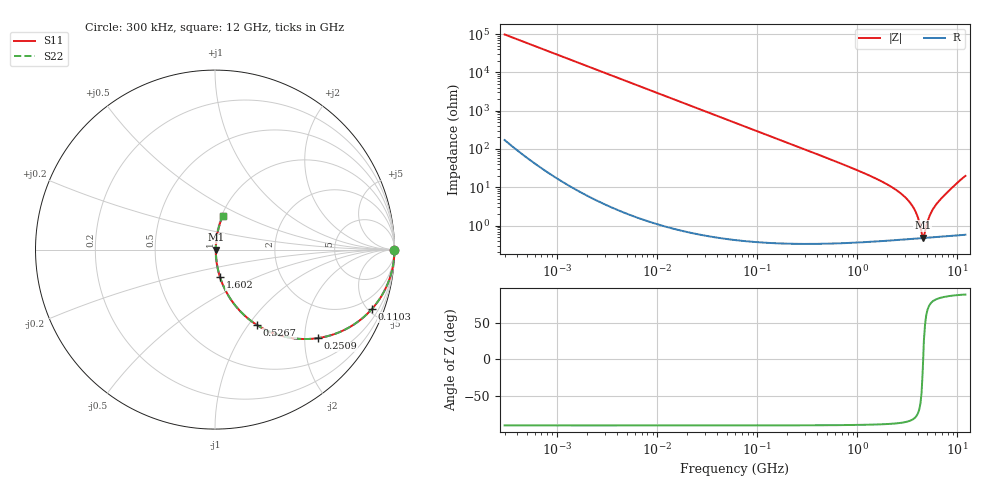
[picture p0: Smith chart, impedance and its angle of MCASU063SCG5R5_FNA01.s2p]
! MCASU063SCG5R5_FNA01  S-PARAMETER MODEL  ( General Type )
! Model Generated by TAIYO YUDEN Corporation (http://www.ty-top.com)
! Version 1.0
! TAIYO YUDEN Control No. 130801
! Copyright(c) 2013 TAIYO YUDEN CO.,LTD. All Rights Reserved.
! Product Description (link to TY-COMPAS)
! https://ds.yuden.co.jp/TYCOMPAS/or/detail?pn=MCASU063SCG5R5DFNA01&u=M
! Products Name : Multilayer Ceramic Capacitors
! Characteristics :
!  Capacitance : 5.5 pF , Rated Voltage : 50V , TCC : CG / C0G
!  Case Size : 0.6 x 0.3 / 0.024 x 0.012 [mm/inch] , Thickness : 0.3 / 0.012 [mm/inch]
!  (Conditions: Temperature = 25 degC , DC Bias Current/Voltage = 0A / 0V)
! External Node Assignments :
!  1  o---| |---o  2
! GND o---------o GND
! Frequency Range : 0.3MHz  -  12000MHz  [ 401 STEP ]
# MHz S RI R 50
! Freq[MHz].  S11 Real  S11 Imag  S21 Real  S21 Imag  S12 Real  S12 Imag  S22 Real  S22 Imag
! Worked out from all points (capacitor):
!   401 points, 300 kHz to 12 GHz, reference 50 ohm
!   read as one part in series: C = 5.44 pF near 316.3 kHz
!   lowest |Z| = 488 mohm at 4.503 GHz (marker M1)
!   series resonance near 4.543 GHz, so ESL is about 230 pH
!   S11 on the Smith chart (normalised r, x): 300 kHz: open; 110.3 MHz: 1.01, -5.30; 250.9 MHz: 1.01, -2.33; 526.7 MHz: 1.01, -1.10; 1.602 GHz: 1.01, -0.32; 12 GHz: 1.01, +0.40
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0.3  1 -0.00102  2.85e-06 0.00102  2.85e-06 0.00102  1 -0.00102
1.769972  1 -0.00605  3.92e-05 0.00605  3.92e-05 0.00605  1 -0.00605
10.44266  0.9987 -0.0356  0.00128 0.0356  0.00128 0.0356  0.9987 -0.0356
27.82928  0.991 -0.0942  0.00901 0.0942  0.00901 0.0942  0.991 -0.0942
60  0.9595 -0.1967  0.0405 0.1967  0.0405 0.1967  0.9595 -0.1967
110.3493  0.8751 -0.3299  0.1249 0.3299  0.1249 0.3299  0.8751 -0.3299
250.8588  0.5749 -0.4929  0.4251 0.4929  0.4251 0.4929  0.5749 -0.4929
353.9943  0.4036 -0.4886  0.5964 0.4886  0.5964 0.4886  0.4036 -0.4886
526.7124  0.2326 -0.4194  0.7674 0.4194  0.7674 0.4194  0.2326 -0.4194
871.3074  0.0974 -0.2911  0.9026 0.2911  0.9026 0.2911  0.0974 -0.2911
1602.47  0.0285 -0.1548  0.9715 0.1548  0.9715 0.1548  0.0285 -0.1548
2088.533  0.016 -0.1084  0.984 0.1084  0.984 0.1084  0.016 -0.1084
2795.104  0.00846 -0.0643  0.9915 0.0643  0.9915 0.0643  0.00846 -0.0643
3454.93  0.00573 -0.0354  0.9943 0.0354  0.9943 0.0354  0.00573 -0.0354
3944.255  0.00492 -0.0182  0.9951 0.0182  0.9951 0.0182  0.00492 -0.0182
4385.161  0.00471 -0.0046  0.9953 0.0046  0.9953 0.0046  0.00471 -0.0046
4502.883  0.00472 -0.00117  0.9953 0.00117  0.9953 0.00117  0.00472 -0.00117
4747.894  0.00479 0.00524  0.9952 -0.00524  0.9952 -0.00524  0.00479 0.00524
5420.343  0.00532 0.0204  0.9947 -0.0204  0.9947 -0.0204  0.00532 0.0204
6188.031  0.00636 0.0363  0.9936 -0.0363  0.9936 -0.0363  0.00636 0.0363
8732.115  0.0141 0.0929  0.9859 -0.0929  0.9859 -0.0929  0.0141 0.0929
12000  0.043 0.1888  0.957 -0.1888  0.957 -0.1888  0.043 0.1888
